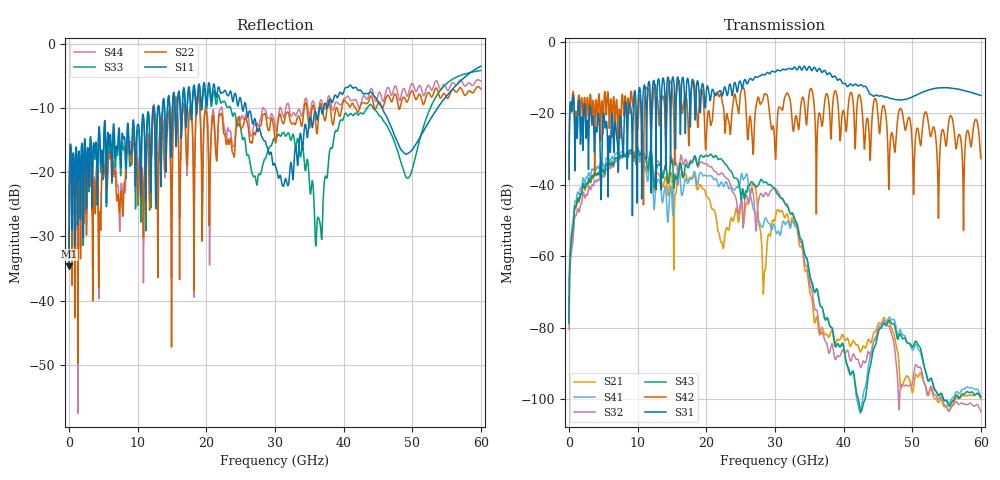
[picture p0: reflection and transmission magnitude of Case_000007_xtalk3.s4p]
! Info: Touchstone file created by circ.  Input file=CasetestDOE_NRZ_template_000007.circ
# Hz S RI R 50
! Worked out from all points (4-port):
!   6000 points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, 10 MHz to 60 GHz, reference 50 ohm
!   strongest paths, dB at 10 MHz, 15.01 GHz, 30.01 GHz, 45.01 GHz, 60 GHz:
!     S31: -38.4, -10.7, -8.4, -15.0, -15.0
!     S42: -38.5, -13.1, -30.5, -20.6, -32.6
!     S43: -78.7, -33.3, -41.3, -81.6, -99.4
!     S32: -80.4, -32.8, -40.8, -80.4, -103.5
!     S41: -77.7, -44.7, -52.0, -80.6, -99.6
!     S21: -78.9, -38.4, -49.6, -79.1, -100.1
!   lowest |S11| = -34.7 dB at 10 MHz (marker M1), VSWR 1.04, Z = 51.2 + j1.44 ohm
!   |S11| at or under -10 dB: start of sweep to 12.22 GHz; 25.81 GHz to 36.48 GHz (10.67 GHz wide, 34.3 % of centre); 45.63 GHz to 53.66 GHz (8.028 GHz wide, 16.2 % of centre)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
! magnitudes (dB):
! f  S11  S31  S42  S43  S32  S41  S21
! 10 MHz  -34.7  -38.4  -38.5  -78.7  -80.4  -77.7  -78.9
! 1.89 GHz  -15.6  -21.9  -16.3  -41.6  -44.4  -39.9  -42.0
! 9.9 GHz  -13.1  -42.5  -21.9  -29.3  -29.7  -30.0  -30.8
! 28.44 GHz  -15.1  -9.2  -14.6  -39.3  -42.9  -49.9  -65.0
! 30.16 GHz  -19.3  -8.2  -30.1  -41.9  -41.2  -53.4  -48.0
! 36.71 GHz  -10.1  -8.1  -21.8  -74.0  -81.7  -74.1  -80.7
! 60 GHz  -3.4  -15.0  -32.6  -99.4  -103.5  -99.6  -100.1
